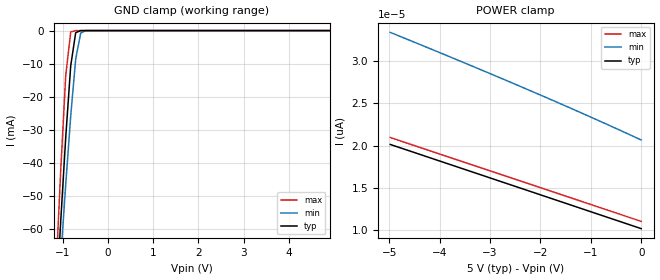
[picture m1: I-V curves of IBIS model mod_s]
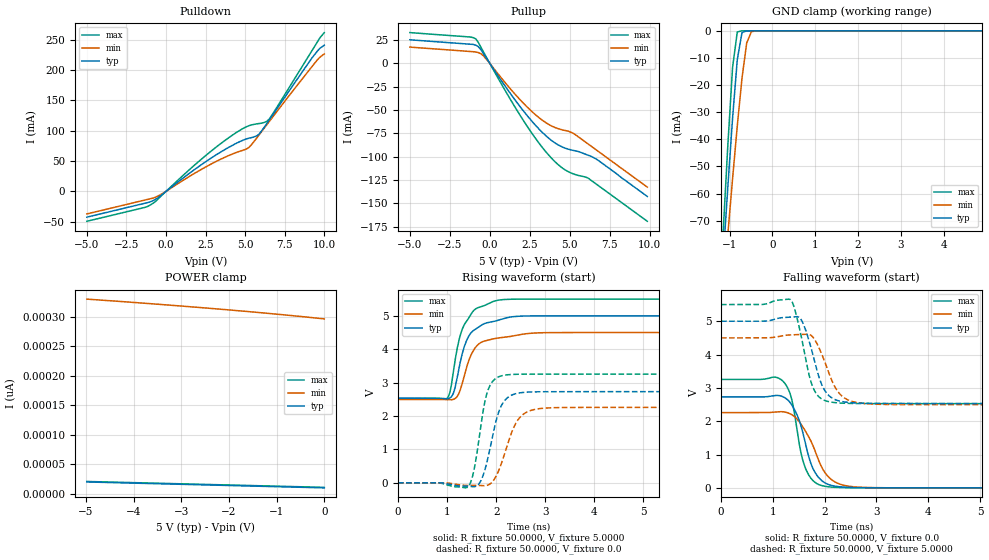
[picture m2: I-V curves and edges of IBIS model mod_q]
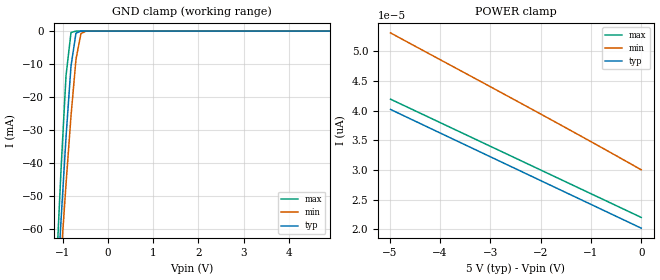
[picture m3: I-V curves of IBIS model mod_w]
| IBIS (I/O, Buffer, Information, Specification) Model, officially
| electronic behavioral standard for Buffer structures of digital pins.
[IBIS ver]  4.0
[File name] m95m02ef_5v0_dfn8.ibs
[File Rev]  1.0
[Date]   21 Jan 2026
[Source]   CAD & Design Services (Catania) - STMicroelectronics
[Notes]
   (Note1)  This IBIS model includes DFN8 Package parasitic data
   (Note2)  This IBIS model considers: VCC=5.00(TYP), 4.50(MIN), 5.50(MAX)
   (Note3)  This IBIS model has some Notes about the non-monotonicity
   of the I-V curves, but they are not indicative of problems
   inside the model;
[Disclaimer]
   Customers are solely responsible for all aspects of their
   own product designs or applications using this IBIS Model.
   STMicroelectronics assumes no liability for Custmer Designs
   and applications associated to this IBIS Model.
   In the use of this IBIS Model Customer shall not modify,
   disassemble, alter this Model in whole or in part.
   If Customers do not accept these terms, the IBIS Model
   may not be used. For any problems or modifications please
   contact STMicroelectronics (www.st.com).
[Copyright] (c) 2026 STMicroelectronics
|   Component M95M02EF
[Component] M95M02EF
[Manufacturer] STMicroelectronics
[Package]
| variable   typ   min   max
R_pkg   0.0   0.0   0.0
L_pkg   0.0H   0.0H   0.0H
C_pkg   0.0F   0.0F   0.0F
[Pin]  signal_name   model_name   R_pin   L_pin   C_pin
1   SN   mod_s   0.0   0.0   0.0
2   Q   mod_q   0.0   0.0   0.0
3   WN   mod_w   0.0   0.0   0.0
4   GND   GND   0.0   0.0   0.0
5   D   mod_d   0.0   0.0   0.0
6   C   mod_c   0.0   0.0   0.0
7   H   mod_h   0.0   0.0   0.0
8   VCC   POWER   0.0   0.0   0.0
[Package Model]  182694_DFN8   | also called 182694_MLP_2x3
[Define Package Model]  182694_DFN8
[Manufacturer]  STMicroelectronics
[OEM]  STMicroelectronics
[Description]  8 pin MLP 2x3
[Number Of Pins]  8
[Pin Numbers]
|Pin Num   Terminal Name
1   | net1
2   | net2
3   | net3
4   | net4_GND
5   | net5
6   | net6
7   | net7
8   | net8_VDD
[Model Data]
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[End Model Data]
[End Package Model]
| Models and submodels in the file (6): mod_s (Input), mod_q (I/O), mod_w (Input), mod_d (Input), mod_c (Input), mod_h (Input)
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|   Model mod_s
[Model]   mod_s
Model_type Input
Vinl   =   1.500V
Vinh   =   3.500V
C_comp   3.207pF   3.063pF   3.358pF
[Temperature Range]  25.0000   85.0000   -40.0000
[Voltage Range]   5.0000V   4.5000V   5.5000V
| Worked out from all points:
|   GND clamp passes 1 mA (typ) near -0.71 V on its own axis
[GND_clamp]
|Voltage   I(typ)   I(min)   I(max)
-5V       -1.086A    -942.6mA   -1.312A
-1.15V    -83.9mA    -91.32mA   -74.15mA
-1.04V    -57.37mA   -68.53mA   -41.97mA
-930mV    -32.19mA   -46.45mA   -13.5mA
-820mV    -10.62mA   -25.76mA   -415.4uA
-710mV    -636.4uA   -8.601mA   -1.855uA
-600mV    -9.649uA   -753uA     -7.81nA
-490mV    -133.7nA   -23.68uA   -35.54pA
4.9V      9.933pA    21.76pA    9.8pA
[POWER_clamp]
|Voltage   I(typ)   I(min)   I(max)
-4.98V    20.14pA    33.44pA    20.96pA
-3.54V    17.25pA    29.9pA     18.08pA
-2.22V    14.59pA    26.57pA    15.44pA
-1.08V    12.3pA     23.59pA    13.16pA
0V        10.13pA    20.66pA    11pA
|   Model mod_q
[Model]   mod_q
Model_type I/O
Polarity   Non-Inverting
Enable   Active-Low
Vinl   =   1.500V
Vinh   =   3.500V
Vmeas  =   2.500V
Cref   =   30pF
C_comp   3.856pF   3.687pF   4.037pF
[Temperature Range]  25.0000   85.0000   -40.0000
[Voltage Range]   5.0000V   4.5000V   5.5000V
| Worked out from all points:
|   slope of the pulldown table from 0 to 0.75 V, typ, clamps not added: 48.6 ohm
|   slope of the pullup table from 0 to 0.75 V, typ, clamps not added: 39.1 ohm
|   GND clamp passes 1 mA (typ) near -0.71 V on its own axis
|   rising waveform, R_fixture 50.0000, V_fixture 5.0000: 20-80 % time 309ps typ, 312ps min, 320ps max; typ from 2.53 V to 5 V
|   rising waveform, R_fixture 50.0000, V_fixture 0.0: 20-80 % time 268ps typ, 335ps min, 216ps max; typ from 0 V to 2.73 V
|   falling waveform, R_fixture 50.0000, V_fixture 0.0: 20-80 % time 317ps typ, 420ps min, 243ps max; typ from 2.73 V to 0 V
|   falling waveform, R_fixture 50.0000, V_fixture 5.0000: 20-80 % time 285ps typ, 332ps min, 253ps max; typ from 5 V to 2.53 V
[Pulldown]
|Voltage   I(typ)   I(min)   I(max)
-5V       -42.43mA   -37.12mA   -49.24mA
-1V       -17.27mA   -12.12mA   -22.55mA
-360mV    -7.533mA   -5.634mA   -8.985mA
2.84V     54.74mA    44.98mA    66.19mA
4.28V     77.13mA    62.54mA    94.24mA
5.24V     87.76mA    72.47mA    108.3mA
5.88V     94.47mA    93.11mA    111.9mA
6.36V     111.6mA    109.6mA    115.4mA
6.84V     129.9mA    126mA      131.8mA
9.24V     220.7mA    206.3mA    232.8mA
9.72V     235.9mA    221.2mA    253.1mA
10V       241mA      226.7mA    261.9mA
[Pullup]
|Voltage   I(typ)   I(min)   I(max)
-5V       25.43mA    17.62mA    33.14mA
-880mV    19.62mA    12.32mA    26.43mA
-720mV    18.03mA    11.68mA    22.47mA
-400mV    10.51mA    8.209mA    12.43mA
2V        -48.7mA    -40.85mA   -58.52mA
2.96V     -68.22mA   -56.52mA   -82.78mA
3.92V     -83.33mA   -67.48mA   -102.7mA
4.56V     -89.71mA   -71.27mA   -112.4mA
5.2V      -93.09mA   -74.65mA   -118.2mA
6V        -97.41mA   -84.48mA   -121.7mA
6.64V     -102.3mA   -92.48mA   -129.1mA
9.84V     -142.5mA   -132.5mA   -169.1mA
[GND_clamp]
|Voltage   I(typ)   I(min)   I(max)
-5V       -1.086A    -869.4mA   -1.312A
-1.15V    -83.9mA    -95.64mA   -74.15mA
-1.04V    -57.37mA   -74.82mA   -41.97mA
-930mV    -32.19mA   -54.5mA    -13.5mA
-820mV    -10.62mA   -35.05mA   -415.4uA
-710mV    -636.4uA   -17.42mA   -1.855uA
-600mV    -9.649uA   -4.458mA   -7.81nA
-490mV    -133.7nA   -325.1uA   -35.54pA
-270mV    -27.92pA   -559nA     -546.7fA
4.9V      9.933pA    299.9pA    9.8pA
[POWER_clamp]
|Voltage   I(typ)   I(min)   I(max)
-4.98V    20.14pA    330pA      20.96pA
-4.2V     18.57pA    325.6pA    19.4pA
-3.3V     16.76pA    320.2pA    17.6pA
-2.7V     15.56pA    316.4pA    16.4pA
-1.92V    13.99pA    311.2pA    14.84pA
-900mV    11.94pA    303.8pA    12.8pA
-540mV    11.22pA    301pA      12.08pA
0V        10.13pA    296.5pA    11pA
[Ramp]
| variable   typ   min   max
dV/dt_r   1.6370/0.2930n   1.3541/0.3722n   1.9520/0.2357n
dV/dt_f   1.4806/0.3050n   1.2034/0.3549n   1.7836/0.2669n
R_load = 50.0000
[Rising Waveform]
R_fixture= 50.0000
V_fixture= 5.0000
V_fixture_min= 4.5000
V_fixture_max= 5.5000
|time   V(typ)   V(min)   V(max)
0s        2.532V     2.494V     2.526V
1.01ns    2.517V     2.487V     2.547V
1.06ns    2.542V     2.484V     2.726V
1.15ns    2.78V      2.512V     3.543V
1.25ns    3.484V     2.709V     4.314V
1.35ns    4.075V     3.205V     4.732V
1.59ns    4.611V     4.074V     5.215V
2.03ns    4.863V     4.334V     5.465V
2.97ns    5V         4.494V     5.5V
10ns      5V         4.5V       5.5V
[Rising Waveform]
R_fixture= 50.0000
V_fixture= 0.0
V_fixture_min= 0.0
V_fixture_max= 0.0
|time   V(typ)   V(min)   V(max)
0s        5.727nV    192.7nV    4.528nV
1.44ns    -102.7mV   -80.41mV   -97.48mV
1.54ns    -118.8mV   -75.69mV   324.9mV
1.66ns    -10.91mV   -79.46mV   1.403V
1.82ns    669.2mV    -74.64mV   2.716V
2ns       1.869V     201.8mV    3.133V
2.14ns    2.397V     724.2mV    3.215V
2.44ns    2.682V     1.877V     3.25V
2.86ns    2.725V     2.216V     3.253V
10ns      2.728V     2.257V     3.253V
[Falling Waveform]
R_fixture= 50.0000
V_fixture= 0.0
V_fixture_min= 0.0
V_fixture_max= 0.0
|time   V(typ)   V(min)   V(max)
0s        2.728V     2.257V     3.253V
1.21ns    2.723V     2.281V     3.177V
1.37ns    2.478V     2.19V      2.619V
1.53ns    1.931V     1.942V     1.149V
1.63ns    1.325V     1.699V     588.8mV
1.79ns    529.8mV    1.207V     194.5mV
1.99ns    164.5mV    492.3mV    51.43mV
2.27ns    34.74mV    125.7mV    10.81mV
2.73ns    4.243mV    15.98mV    1.047mV
10ns      51.18nV    199.1nV    21.01nV
[Falling Waveform]
R_fixture= 50.0000
V_fixture= 5.0000
V_fixture_min= 4.5000
V_fixture_max= 5.5000
|time   V(typ)   V(min)   V(max)
0s        5V         4.5V       5.5V
1.34ns    5.123V     4.59V      5.649V
1.42ns    5.13V      4.595V     5.374V
1.54ns    5.063V     4.601V     4.603V
1.76ns    4.074V     4.544V     3.073V
1.92ns    3.189V     4.099V     2.691V
2.1ns     2.743V     3.369V     2.58V
2.36ns    2.583V     2.722V     2.54V
2.82ns    2.539V     2.524V     2.528V
10ns      2.532V     2.494V     2.526V
|   Model mod_w
[Model]   mod_w
Model_type Input
Vinl   =   1.500V
Vinh   =   3.500V
C_comp   3.207pF   3.063pF   3.358pF
[Temperature Range]  25.0000   85.0000   -40.0000
[Voltage Range]   5.0000V   4.5000V   5.5000V
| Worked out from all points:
|   GND clamp passes 1 mA (typ) near -0.71 V on its own axis
[GND_clamp]
|Voltage   I(typ)   I(min)   I(max)
-5V       -1.086A    -942.6mA   -1.312A
-1.15V    -83.9mA    -91.32mA   -74.15mA
-1.04V    -57.37mA   -68.53mA   -41.97mA
-930mV    -32.19mA   -46.45mA   -13.5mA
-820mV    -10.62mA   -25.76mA   -419.8uA
-710mV    -639.4uA   -8.604mA   -2.115uA
-600mV    -9.894uA   -755.1uA   -9.088nA
-490mV    -137.6nA   -23.91uA   -42.86pA
4.9V      19.79pA    31.94pA    19.6pA
[POWER_clamp]
|Voltage   I(typ)   I(min)   I(max)
-4.98V    40.19pA    53.1pA     41.92pA
-1.98V    28.14pA    39.34pA    29.92pA
-900mV    23.8pA     34.3pA     25.6pA
0V        20.19pA    30.02pA    22pA
